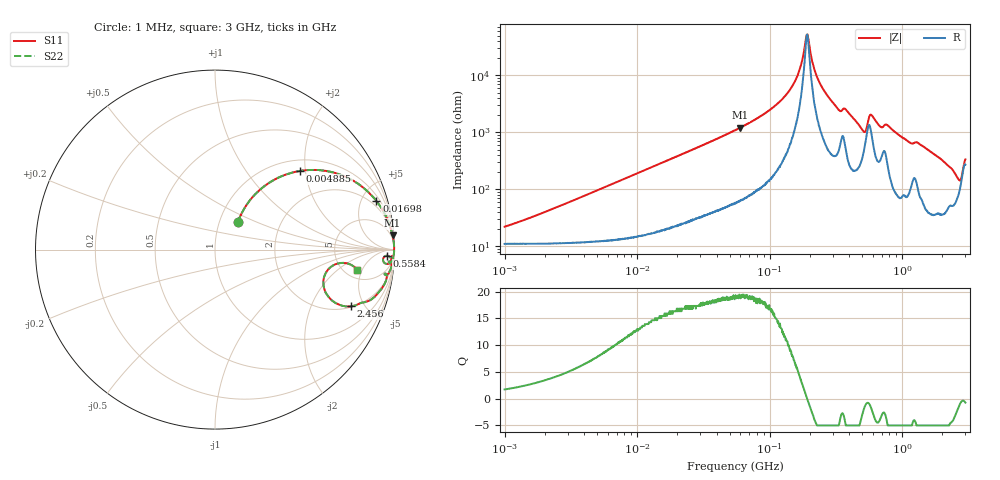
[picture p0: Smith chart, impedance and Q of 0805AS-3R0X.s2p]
!s-Parameter Generated by FASTRON Sdn. Bhd.
!FASTRON P/N : 0805AS-3R0X
!Keysight Technologies: E4991B_MY54100416_A.01.15
!Date: Mon Jun 15 12:58:23 2026
!Version  :Rev01  Mon Jun 15 12:58:23 2026
!Data & Calibration Information:
!Freq  S11  S21  S12  S22
!PortZ  Port1:50+j0  Port2:50+j0
!When reading reference impedance value at option line is always used.
! Remarks : This data is being provided solely for informational purposes.
# Hz S dB R 50
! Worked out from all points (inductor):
!   1601 points, 1 MHz to 3 GHz, reference 50 ohm
!   read as one part in series: L = 3.05 uH near 1.743 MHz
!   highest Q = 19.2 at 60.24 MHz (marker M1), where L = 3.22 uH
!   self-resonance near 191.4 MHz
!   S11 on the Smith chart (normalised r, x): 1 MHz: 1.22, +0.39; 4.885 MHz: 1.24, +1.87; 16.98 MHz: 1.41, +6.47; 558.4 MHz: 27, -22; 2.456 GHz: 2.06, -3.96; 3 GHz: 6.43, -3.95
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1000000  -14.10 50.1  -1.04 -9.8  -1.04 -9.8  -14.10 50.1
3804036  -5.14 47.7  -2.51 -33.1  -2.51 -33.1  -5.14 47.7
4885451  -3.79 42.7  -3.29 -39.8  -3.29 -39.8  -3.79 42.7
1.447069e7  -0.71 19.4  -9.56 -66.8  -9.56 -66.8  -0.71 19.4
1.698367e7  -0.55 16.8  -10.80 -69.6  -10.80 -69.6  -0.55 16.8
5.504702e7  -0.08 5.2  -20.90 -81.8  -20.90 -81.8  -0.08 5.2
6.023535e7  -0.07 4.7  -21.80 -82.3  -21.80 -82.3  -0.07 4.7
1.361705e8  -0.02 1.2  -33.80 -83.5  -33.80 -83.5  -0.02 1.2
1.646891e8  -0.02 0.5  -40.80 -77.8  -40.80 -77.8  -0.02 0.5
1.904091e8  -0.02 0.0  -54.30 -13.2  -54.30 -13.2  -0.02 0.0
2.083556e8  -0.02 -0.3  -45.50 68.4  -45.50 68.4  -0.02 -0.3
2.433181e8  -0.02 -0.8  -36.70 80.5  -36.70 80.5  -0.02 -0.8
3.268837e8  -0.06 -2.1  -28.40 78.2  -28.40 78.2  -0.06 -2.1
3.760477e8  -0.07 -2.2  -28.10 76.7  -28.10 76.7  -0.07 -2.2
5.102796e8  -0.37 -4.8  -20.80 60.8  -20.80 60.8  -0.37 -4.8
5.583748e8  -0.38 -2.0  -25.10 38.0  -25.10 38.0  -0.38 -2.0
5.870266e8  -0.20 -2.5  -26.30 60.0  -26.30 60.0  -0.20 -2.5
7.925923e8  -0.13 -4.4  -22.30 76.5  -22.30 76.5  -0.13 -4.4
1.712864e9  -0.39 -12.9  -13.00 72.3  -13.00 72.3  -0.39 -12.9
2.455801e9  -1.73 -22.7  -7.97 52.3  -7.97 52.3  -1.73 -22.7
2.727913e9  -3.92 -18.3  -7.07 26.8  -7.07 26.8  -3.92 -18.3
3e9  -1.96 -8.0  -12.50 28.0  -12.50 28.0  -1.96 -8.0
